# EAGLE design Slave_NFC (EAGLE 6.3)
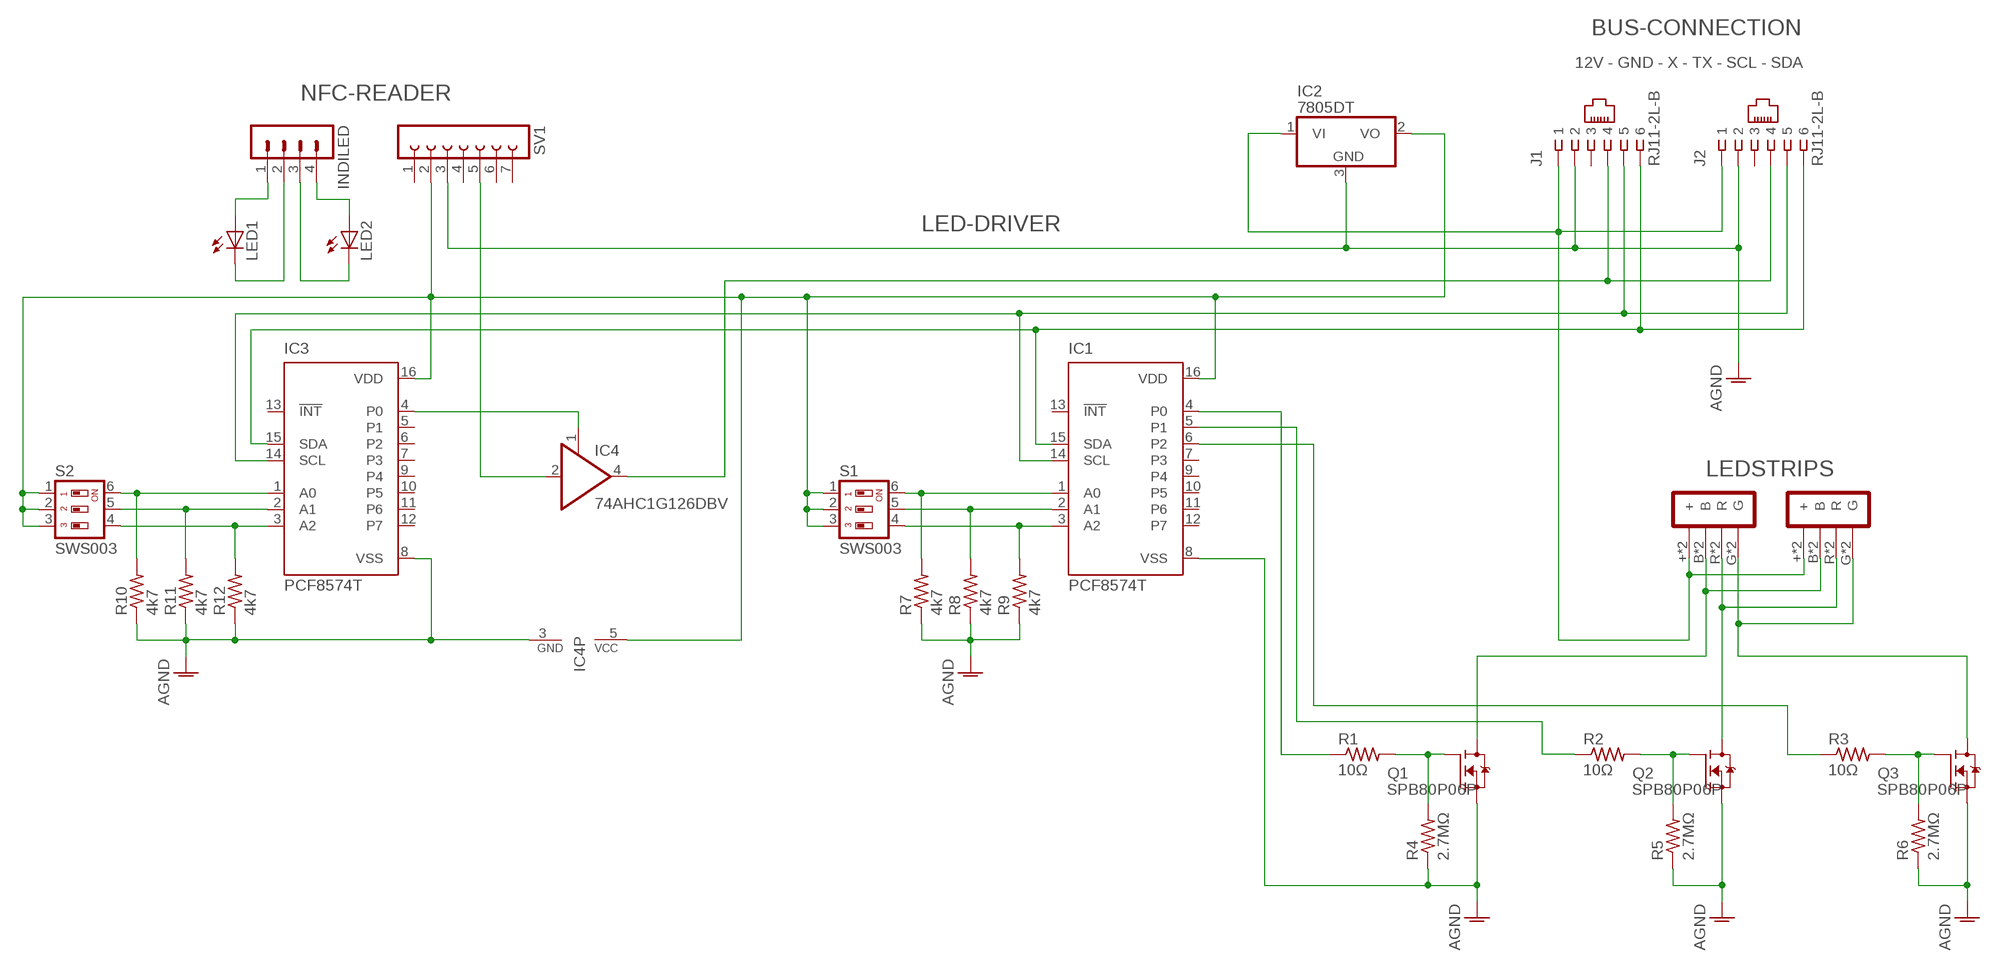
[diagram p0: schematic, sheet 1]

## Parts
IC1  PCF8574T  [SO16W]
IC2  7805DT  [TO252]
IC3  PCF8574T  [SO16W]
IC4  74AHC1G126DBV  [SOT23-5]
INDILED  MA04-1  [MA04-1]
J1  RJ11-2L-B  [RJ11-NO_SHIELD]
J2  RJ11-2L-B  [RJ11-NO_SHIELD]
LED1  LEDB152  [Q62902-B152]
LED2  LEDB152  [Q62902-B152]
Q1  SPB80P06P  [TO263]
Q2  SPB80P06P  [TO263]
Q3  SPB80P06P  [TO263]
R1  10Ω  R-US_R0402  [R0402]
R2  10Ω  R-US_R0402  [R0402]
R3  10Ω  R-US_R0402  [R0402]
R4  2.7MΩ  R-US_R0402  [R0402]
R5  2.7MΩ  R-US_R0402  [R0402]
R6  2.7MΩ  R-US_R0402  [R0402]
R7  4k7  R-US_R0402  [R0402]
R8  4k7  R-US_R0402  [R0402]
R9  4k7  R-US_R0402  [R0402]
R10  4k7  R-US_R0402  [R0402]
R11  4k7  R-US_R0402  [R0402]
R12  4k7  R-US_R0402  [R0402]
S1  SWS003  [SMS-003]
S2  SWS003  [SMS-003]
SV1  FE07-1  [FE07]
U$1  LED_S  [LED_P]
U$2  LED_S  [LED_P]

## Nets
AGND: IC1.8(VSS) IC2.3(GND) IC3.8(VSS) IC4.3(GND) J1.2 J2.2 Q1.2(D) Q2.2(D) Q3.2(D) R4.1 R5.1 R6.1 R7.1 R8.1 R9.1 R10.1 R11.1 R12.1 SV1.3
N$1: IC1.15(SDA) IC3.15(SDA) J1.6 J2.6
N$2: IC4.4(O) J1.4 J2.4
N$3: IC1.14(SCL) J1.5 J2.5
N$4: Q1.1(G) R1.2 R4.2
N$5: Q2.1(G) R2.2 R5.2
N$6: Q3.1(G) R3.2 R6.2
N$7: Q1.3(S) U$1.B U$1.B1(B) U$2.B U$2.B1(B)
N$8: Q2.3(S) U$1.R U$1.R1(R) U$2.R U$2.R1(R)
N$9: Q3.3(S) U$1.G U$1.G1(G) U$2.G U$2.G1(G)
N$10: IC2.1(VI) J1.1 J2.1 U$1.+ U$1.+1(+) U$2.+ U$2.+1(+)
N$11: IC3.1(A0) R10.2 S2.6
N$12: IC1.1(A0) R7.2 S1.6
N$13: IC1.2(A1) R8.2 S1.5
N$14: IC1.3(A2) R9.2 S1.4
N$15: IC3.4(P0) IC4.1(OE)
N$16: IC1.4(P0) R1.1
N$17: IC1.5(P1) R2.1
N$18: IC1.6(P2) R3.1
N$19: IC3.2(A1) R11.2 S2.5
N$20: IC3.3(A2) R12.2 S2.4
N$21: IC1.16(VDD) IC2.2(VO) IC3.16(VDD) IC4.5(VCC) S1.1 S1.2 S1.3 S2.1 S2.2 S2.3 SV1.2
N$22: INDILED.1 LED1.A
N$23: INDILED.4 LED2.A
N$24: INDILED.2 LED1.K(C)
N$25: INDILED.3 LED2.K(C)
N$27: IC4.2(I) SV1.5
Unconnected: IC1.7(P3) IC1.9(P4) IC1.10(P5) IC1.11(P6) IC1.12(P7) IC1.13(!INT) IC3.5(P1) IC3.6(P2) IC3.7(P3) IC3.9(P4) IC3.10(P5) IC3.11(P6) IC3.12(P7) IC3.13(!INT) IC3.14(SCL) J1.3 J2.3 SV1.1 SV1.4 SV1.6 SV1.7

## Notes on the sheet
- BUS-CONNECTION
- 12V - GND - X - TX - SCL - SDA
- NFC-READER
- LED-DRIVER
- LEDSTRIPS

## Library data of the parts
IC1 IC3 = micro-philips:PCF8574: I2C-Bus Remote 8-bit I/O expander http://www.semiconductors.philips.com/acrobat_download/datasheets/PCF8574_4.pdf; MPN: PCF8574T/3,512; OC_FARNELL: 1201255; OC_NEWARK: 70R6870
IC2 = linear:78*: Positive VOLTAGE REGULATOR Source: http://cache.national.com/ds/LM/LM78L05.pdf http://www.fairchildsemi.com/ds/LM/LM7805.pdf
IC4 = 74xx-little-de:74*1G126: Single Bus Buffer Gate With 3-State Outputs
INDILED = con-lstb:MA04-1: PIN HEADER; OC_FARNELL: unknown; OC_NEWARK: unknown
J1 J2 = con-tycoelectronics:RJ11: CORCOM Modular RJ Jacks No Shield Source: www.tycoelectronics.com .. ENG_DS_1654001_1099_RJ_L_0507.pdf; MF: TYCO ELECTRONICS; MPN: RJ11-2L-B; OC_FARNELL: unknown; OC_NEWARK: 83F4463
LED1 LED2 = led:LED: LED
Q1-Q3 = F3205S:SPB80P06P: SIPMOS (R) Power-Transistor P-Channel, Enhancement mode Source: http://www.infineon.com/upload/Document/cmc_upload/documents/011/3685/SPP80P06P.pdf
R1-R12 = rcl:R-US_: RESISTOR, American symbol
S1 S2 = smd-special:SWS003: SMD Dip Switch 3 pol.
SV1 = con-lsta:FE07-1: FEMALE HEADER; OC_FARNELL: unknown; OC_NEWARK: unknown
U$1 U$2 = Onboard_LEDstrip:LED_S

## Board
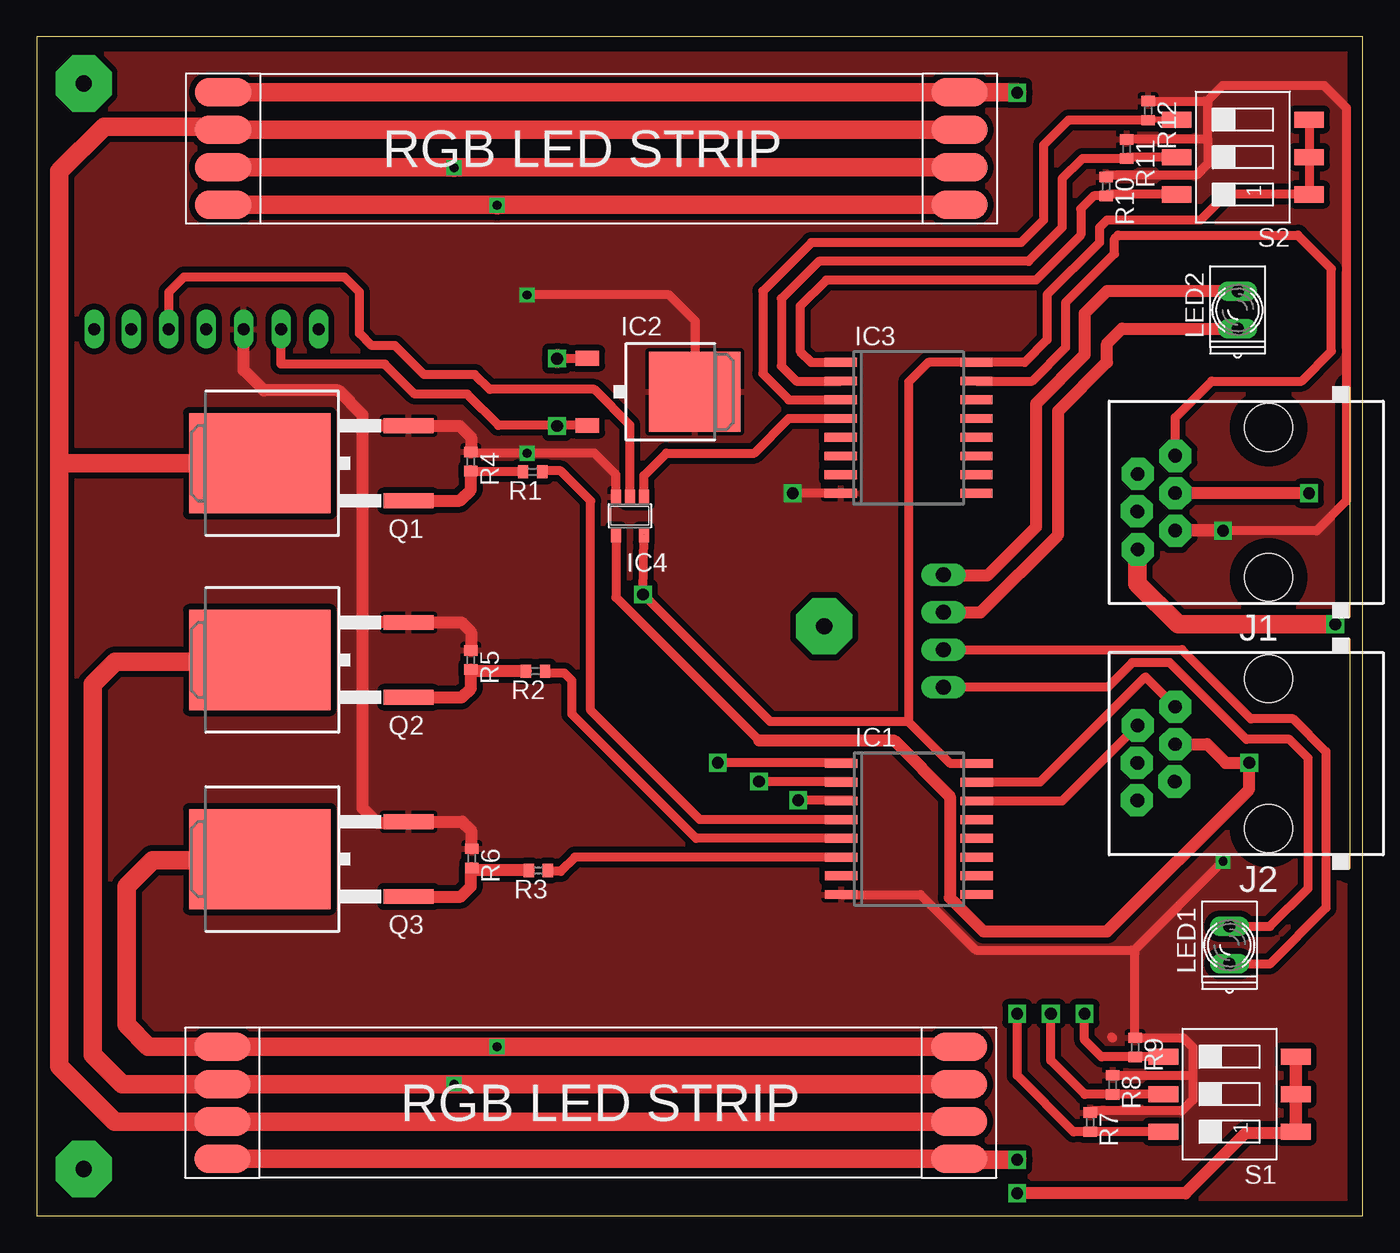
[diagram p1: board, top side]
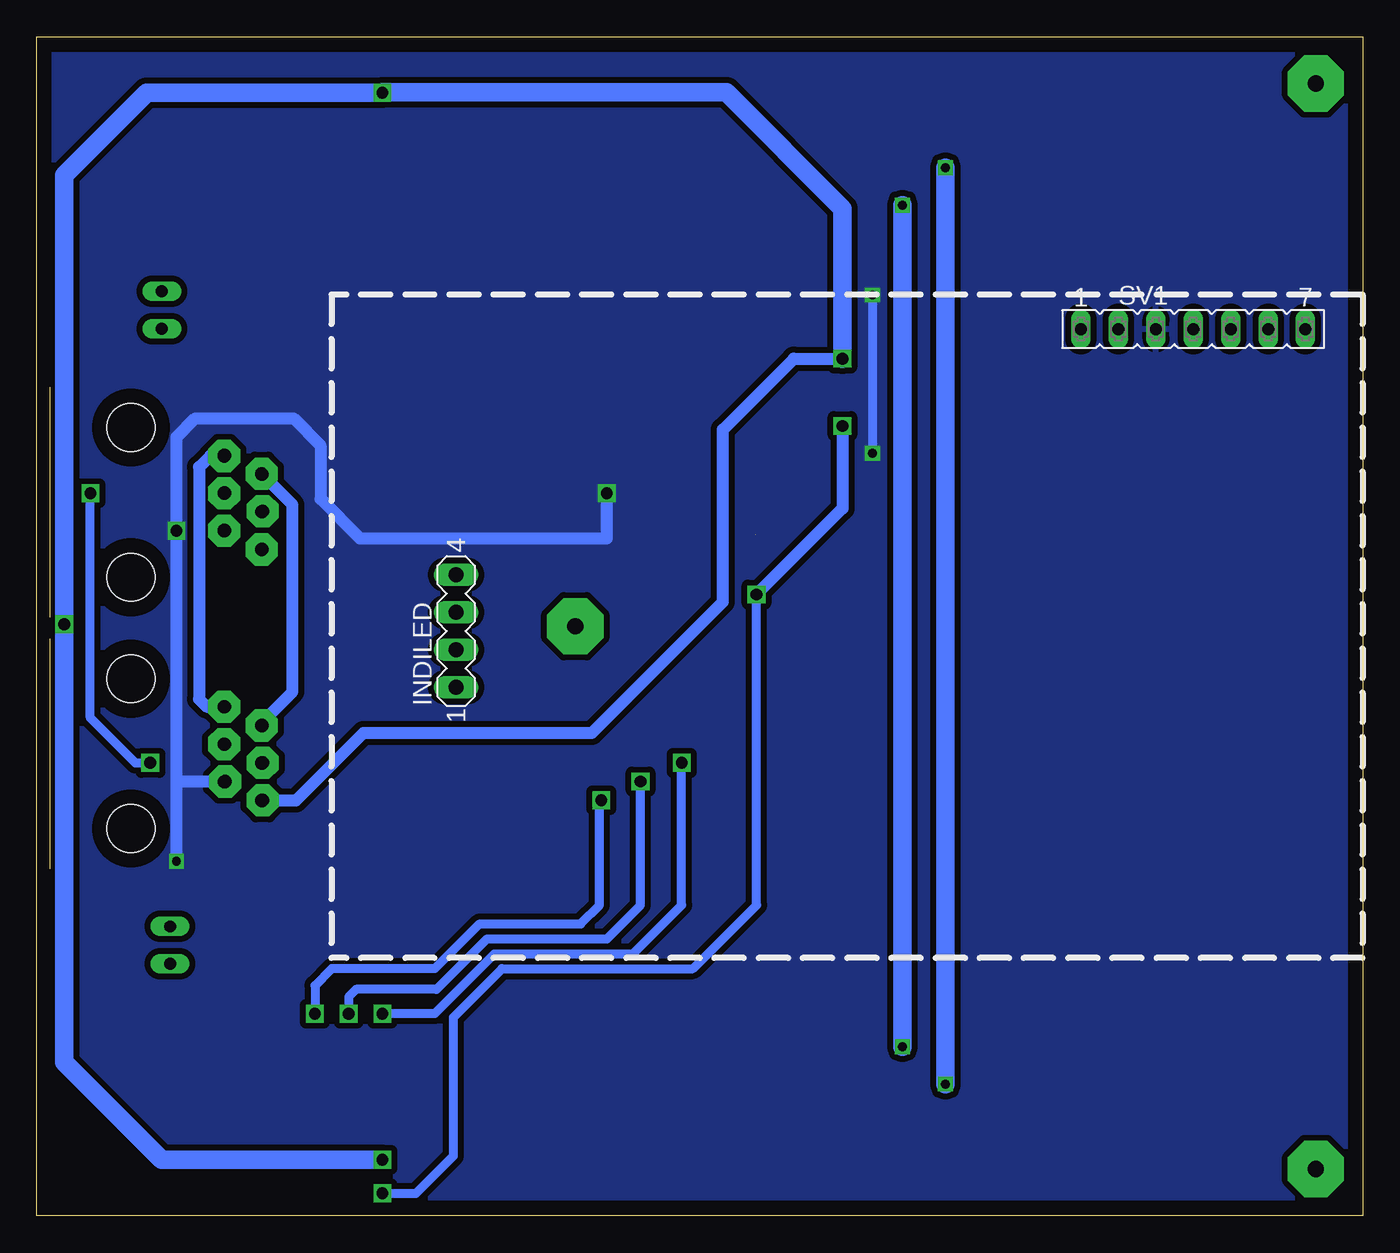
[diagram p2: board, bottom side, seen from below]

Size 90 x 80 mm. Coordinates in mm from the lower left corner, seen from the top.
Outline: 0,0 90,0 90,80 0,80 0,0
Copper layers (1*16): Top 0.035mm / dielectric 1.5mm / Bottom 0.035mm
Design rules "default": minimum track width 10mil, minimum drill 24mil, track to track 8mil, track to pad 8mil, pad to pad 8mil, via to via 8mil, smd to smd 8mil, copper to edge 40mil, drill to drill 8mil, minimum pad ring 10mil, minimum via ring 8mil, stop-mask expansion 4mil, vias tented up to drill 0mil, thermal gap 10mil

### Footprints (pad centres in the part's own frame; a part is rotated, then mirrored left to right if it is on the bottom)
SO16W = smd 0.6 x 2.2: 1 -4.445,-4.6; 2 -3.175,-4.6; 3 -1.905,-4.6; 4 -0.635,-4.6; 5 0.635,-4.6; 6 1.905,-4.6; 7 3.175,-4.6; 8 4.445,-4.6; 9 4.445,4.6; 10 3.175,4.6; 11 1.905,4.6; 12 0.635,4.6; 13 -0.635,4.6; 14 -1.905,4.6; 15 -3.175,4.6; 16 -4.445,4.6
TO252 = smd 1 x 1.6: 1 -2.28,-4.8; 2 2.28,-4.8 | smd 5.4 x 6.2: 3 0,2.5
SOT23-5 = smd 0.69 x 0.99: 1 -0.95,-1.29; 2 0,-1.29; 3 0.95,-1.29; 4 0.95,1.3; 5 -0.95,1.3
MA04-1 = drill 1.016 long: 1 -3.81,0; 2 -1.27,0; 3 1.27,0; 4 3.81,0
RJ11-NO_SHIELD = drill 0.9 pad 1.4: 1 -3.175,8.89; 2 -1.905,6.35; 3 -0.635,8.89; 4 0.635,6.35; 5 1.905,8.89; 6 3.175,6.35 | hole 3.251: -5.08,0; 5.08,0
Q62902-B152 = drill 0.813 long: A 1.27,0; K -1.27,0
TO263 = smd 1 x 3.4: 1 -2.54,-6.6; 2 2.54,-6.6 | smd 6.8 x 9.6: 3 0,3.5
R0402 = smd 0.7 x 0.9: 1 -0.65,0; 2 0.65,0
SMS-003 = smd 1.092 x 2.007: 1 -2.54,-4.496; 2 0,-4.496; 3 2.54,-4.496; 4 2.54,4.496; 5 0,4.496; 6 -2.54,4.496
FE07 = drill 0.813 long: 1 -7.62,0; 2 -5.08,0; 3 -2.54,0; 4 0,0; 5 2.54,0; 6 5.08,0; 7 7.62,0
LED_P = smd 3.81 x 1.93: + -24.13,3.81; +1 25.87,3.81; B -24.13,1.27; B1 25.87,1.27; G -24.13,-3.81; G1 25.87,-3.81; R -24.13,-1.27; R1 25.87,-1.27

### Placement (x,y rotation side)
IC1  59.2,26.25 270 top
IC2  42.17,55.91 270 top
IC3  59.18,53.47 270 top
IC4  40.26,47.5 180 top
INDILED  61.54,39.68 90 bottom
J1  83.61,48.41 90 top
J2  83.61,31.36 90 top
LED1  80.96,18.36 90 top
LED2  81.51,61.47 90 top
Q1  18.63,51.06 90 top
Q2  18.64,37.72 90 top
Q3  18.64,24.2 90 top
R1  33.66,50.48 180 top
R2  33.85,36.96 180 top
R3  34.04,23.43 180 top
R4  29.46,51.18 270 top
R5  29.46,37.72 270 top
R6  29.53,24.26 270 top
R7  71.5,6.35 270 top
R8  73.03,8.89 270 top
R9  74.55,11.43 270 top
R10  72.58,69.85 270 top
R11  73.98,72.39 270 top
R12  75.44,74.99 270 top
S1  80.96,8.26 90 top
S2  81.87,71.84 90 top
SV1  11.5,60.17 0 bottom
U$1  36.78,72.42 0 top
U$2  38.47,7.67 180 top

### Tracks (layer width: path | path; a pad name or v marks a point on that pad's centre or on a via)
AGND  (via drill 0.6, 0.8)
  Top 0.406: 72.58,70.61 R10.1
  Top 0.61: R12.1 79.3,75.64 79.5,75.44 | 79.5,73.04 R11.1 | 79.5,73.04 79.5,71.37 78.74,70.61 72.69,70.61 R10.1 | 79.5,73.04 79.5,75.44 | v80.52,46.48 86.87,46.48 88.9,48.51 88.9,75.18 87.38,76.71 80.52,76.71 79.5,75.69 79.5,75.44 | 78.49,9.4 78.49,11.43 77.84,12.08 R9.1 74.55,17.84 74.36,18.03 | 78.49,9.4 78.49,7.87 77.72,7.11 71.61,7.11 R7.1 | R8.1 78.34,9.54 78.49,9.4 | 73.01,12.08 72.96,12.13 | IC4.3 39.31,50.29 37.85,51.75 v33.27,51.75 29.54,51.75 R4.1 | IC1.8 59.99,21.8 63.75,18.03 74.49,18.03 v80.52,24.07 | IC2.3 44.7,55.91 44.7,60.71 42.93,62.48 v33.27,62.48 | IC3.8 v51.31,49.02
  Top 0.813: R6.1 29.46,24.97 29.46,26.16 28.88,26.74 Q3.2 25.17,26.67 23.11,26.67 22.1,27.69 22.1,40.13 | R5.1 29.46,39.62 28.83,40.26 Q2.2 22.23,40.26 22.1,40.13 | R4.1 29.46,52.83 28.69,53.6 Q1.2 22.11,53.6 22.1,52.83 | 22.1,52.83 22.1,40.13 | 22.1,52.83 22.1,54.36 20.45,56.01 15.43,56.01 14.03,57.4 SV1.3 | IC2.3 44.96,56.21 | v80.52,46.48 77.28,46.48 | v80.5,46.51 J1.2
  Bottom 0.61: v33.27,62.48 v33.27,51.75
  Bottom 0.813: 80.52,29.46 v80.52,46.48 | J2.2 80.51,29.45 80.52,29.46 | v80.5,46.51 v80.52,46.48 | v80.52,46.48 80.52,52.83 79.25,54.1 72.58,54.1 70.74,52.26 70.74,48.64 68.07,45.97 51.31,45.97 v51.31,49.02 | v80.52,24.07 80.52,29.46
  pour Bottom (isolate 0.406): 0.13,80.01 89.98,80.01 89.98,0 0,0 0,80.01
  pour Top (isolate 0.406): 0,80.01 89.92,80.01 89.92,0 0,0
N$1  (via drill 0.9 pad 2.18)
  Top 0.61: IC3.15 67.56,56.64 69.85,58.93 69.85,61.98 73.15,65.28 73.15,66.29 73.41,66.55 85.6,66.55 87.88,64.26 87.88,58.67 85.85,56.64 79.76,56.64 77.28,54.17 77.28,51.56 J1.6 | v77.27,34.54 J2.6 | v77.28,34.54 75.25,36.58 68.09,29.42 IC1.15
  Bottom 0.813: J2.6 v77.27,34.54 v77.28,34.54 78.49,34.54 78.99,35.05 78.99,50.8 78.21,51.59 J1.6
N$2  (via drill 0.8, 0.9 pad 2.18)
  Top 0.61: IC4.4 39.31,41.97 49.02,32.26
  Top 0.813: 49.02,32.26 58.17,32.26 61.98,28.45 61.98,21.59 64.26,19.3 72.64,19.3 82.3,28.96 v82.3,30.73 80.71,30.73 79.44,32 v77.28,32 J2.4 | v86.36,49.02 77.28,49.02 J1.4
  Bottom 0.61: v86.36,49.02 86.36,33.78 83.31,30.73 v82.3,30.73
  Bottom 0.813: 77.28,49.02 J1.4
N$3
  Top 0.61: IC1.14 69.61,28.15 J2.5
  Bottom 0.813: J2.5 74.72,33.48 72.64,35.56 72.64,48.24 J1.5
N$4
  Top 0.61: R1.2 29.51,50.48
  Top 0.813: Q1.1 28.71,48.52 29.46,49.28 R4.2 29.51,50.48
N$5
  Top 0.813: Q2.1 28.83,35.18 29.46,35.81 R5.2 29.58,36.96 R2.2
N$6
  Top 0.813: Q3.1 28.77,21.66 29.46,22.35 29.46,23.54 R6.2 29.7,23.43 R3.2
N$7
  Top 1.27: U$2.B U$2.B1 5.29,6.4 1.52,10.16 1.52,51.05 | 12.06,73.69 U$1.B 13.21,73.69 | U$1.B1 13.21,73.69 | 1.52,51.05 1.52,70.87 4.57,73.91 12.98,73.91 13.21,73.69 | Q1.3 1.53,51.06 1.52,51.05
N$8  (via drill 0.6)
  Top 1.27: U$2.R 62.6,9.21 61.91,9.21 61.91,8.94 28.83,8.94 v28.32,8.94 U$2.R1 5.79,8.94 3.81,10.92 3.81,36.07 5.33,37.59 11.68,37.59 11.94,37.34 11.71,37.34 Q2.3 | U$1.R1 U$1.R 28.3,71.14 v28.32,71.12
  Bottom 1.27: v28.32,71.12 v28.32,8.94
N$9  (via drill 0.6)
  Top 1.27: U$2.G v31.24,11.48 30.99,11.48 U$2.G1 7.57,11.48 6.1,12.95 6.1,22.35 7.87,24.13 15.07,24.13 Q3.3 | U$1.G1 U$1.G 31.22,68.61 v31.24,68.58
  Bottom 1.27: v31.24,68.58 v31.24,11.48
N$10  (via drill 0.8)
  Top 0.61: 35.34,58.2 IC2.1
  Top 1.27: U$2.+1 U$2.+ 62.65,3.81 v66.55,3.81 | U$1.+ U$1.+1 66.52,76.22 v66.55,76.2 | J1.1 74.72,42.88 77.47,40.13 v88.14,40.13 | 35.34,58.2 v35.31,58.17
  Bottom 0.813: J2.1 72.4,28.18 67.82,32.77 52.32,32.77 43.43,41.66 43.43,53.34 38.61,58.17 v35.31,58.17
  Bottom 1.27: v66.55,3.81 81.53,3.81 88.14,10.41 v88.14,40.13 88.14,70.61 82.55,76.2 v66.55,76.2 66.52,76.22 43.18,76.22 35.31,68.35 v35.31,58.17
N$11
  Top 0.406: 72.58,69.3 R10.2
  Top 0.61: S2.6 72.68,69.3 R10.2 71.74,69.2 70.87,68.33 70.87,66.55 67.82,63.5 53.59,63.5 51.82,61.72 51.82,58.67 52.58,57.91 IC3.1
N$12  (via drill 0.8)
  Top 0.61: S1.6 71.52,5.71 R7.2 70.37,5.7 66.55,9.53 v66.55,13.72 | IC1.1 55.38,30.73 v46.23,30.73
  Bottom 0.61: v66.55,13.72 62.99,13.72 58.93,17.78 49.53,17.78 46.23,21.08 v46.23,30.73
N$13  (via drill 0.8)
  Top 0.61: S1.5 73.04,8.26 R8.2 71.14,8.24 68.83,10.54 v68.83,13.72 | IC1.2 55.38,29.46 v49.02,29.46
  Bottom 0.61: v68.83,13.72 68.83,14.86 68.33,15.37 62.87,15.37 59.44,18.8 51.31,18.8 49.02,21.08 v49.02,29.46
N$14  (via drill 0.8)
  Top 0.61: S1.4 74.56,10.79 R9.2 72.28,10.78 71.12,11.94 v71.12,13.72 | IC1.3 55.38,28.19 v51.69,28.19
  Bottom 0.61: v71.12,13.72 71.12,15.62 69.98,16.76 62.99,16.76 59.94,19.81 53.09,19.81 51.82,21.08 51.82,28.07 v51.69,28.19
N$15
  Top 0.61: IC4.1 41.21,50.23 42.74,51.75 48.7,51.75 51.05,54.1 IC3.4
N$16
  Top 0.61: IC1.4 45,26.88 37.59,34.29 37.59,48.51 35.56,50.55 34.37,50.55 R1.1
N$17
  Top 0.61: IC1.5 44.75,25.61 36.32,34.04 36.32,36.32 35.81,36.83 34.62,36.83 R2.1
N$18
  Top 0.61: IC1.6 36.53,24.34 35.56,23.37 34.75,23.37 R3.1
N$19
  Top 0.406: 73.98,71.84 R11.2
  Top 0.61: S2.5 74.08,71.84 R11.2 70.98,71.74 69.6,70.36 69.6,67.06 67.31,64.77 53.09,64.77 50.55,62.23 50.55,57.66 51.56,56.64 IC3.2
N$20
  Top 0.406: S2.4 75.44,74.38 R12.2
  Top 0.61: R12.2 70.03,74.34 68.33,72.64 68.33,67.56 66.8,66.04 52.58,66.04 49.28,62.74 49.28,57.15 51.05,55.37 IC3.3
N$21  (via drill 0.8)  (1 unrouted)
  Top 0.61: S2.3 S2.2 S2.1 80.73,69.3 78.99,67.56 72.64,67.56 72.14,67.06 72.14,66.04 68.58,62.48 68.58,59.44 67.06,57.91 IC3.16 60.52,57.91 59.18,56.58 59.18,33.53 | IC2.2 35.31,53.63 | 35.31,53.63 v35.31,53.59 | 35.31,53.63 31.33,53.63 29.21,55.75 25.65,55.75 23.62,57.78 16.57,57.78 SV1.2 | IC4.5 v41.15,42.16 49.78,33.53 59.18,33.53 | IC1.16 62.02,30.69 59.18,33.53
  Top 0.813: 35.35,53.63 v35.31,53.59 | S1.1 S1.2 S1.3 S1.1 85.6,5.59 82.04,5.59 77.98,1.52 v66.55,1.52
  Bottom 0.61: v66.55,1.52 64.26,1.52 61.72,4.06 61.72,13.46 58.42,16.76 45.47,16.76 41.15,21.08 v41.15,42.16
  Bottom 0.813: v35.31,53.59 35.31,48.01 v41.15,42.16
N$22
  Top 0.61: LED1.A 83.7,19.63 86.3,22.23 86.3,31.05 85.03,32.32 82.11,32.32 76.9,37.53 74.36,37.53 72.71,35.88 INDILED.1
N$23
  Top 0.813: LED2.A 72.64,62.74 71.12,61.21 71.12,58.42 67.82,55.12 67.82,46.74 64.52,43.43 61.6,43.43 INDILED.4
N$24
  Top 0.61: INDILED.2 77.73,38.41 82.42,33.72 85.28,33.72 87.5,31.5 87.5,20.89 83.69,17.08 LED1.K
N$25
  Top 0.813: INDILED.3 64.06,40.95 69.34,46.23 69.34,54.61 72.64,57.91 72.64,59.18 73.66,60.2 LED2.K
N$27
  Top 0.61: IC4.2 40.26,53.66 37.85,56.07 30.73,56.07 29.72,57.09 26.29,57.09 24.32,59.05 22.73,59.05 21.91,59.88 21.91,62.67 20.89,63.69 9.97,63.69 8.95,62.67 SV1.5
N$28  (via drill 0.9 pad 2.18)
  other vias: 74.74,33.27
N$29  (via drill 0.9 pad 2.18)
  other vias: 74.68,30.73
N$30  (via drill 0.9 pad 2.18)
  other vias: 77.22,29.46
N$31  (via drill 0.9 pad 2.18)
  other vias: 74.68,28.19
N$32  (via drill 0.9 pad 2.18)
  other vias: 74.74,50.36
N$33  (via drill 0.9 pad 2.18)
  other vias: 74.68,47.82
N$34  (via drill 0.9 pad 2.18)
  other vias: 74.74,45.21
N$35  (via drill 0.9 pad 2.18)
  other vias: 77.28,46.48
N$36  (via drill 0.9 pad 2.18)
  other vias: 77.28,49.02
N$37  (via drill 0.9 pad 2.18)
  other vias: 77.28,51.56
N$38  (via drill 1.1 pad 3.81)
  other vias: 3.17,76.83
N$39  (via drill 1.1 pad 3.81)
  other vias: 3.17,3.17
N$40  (via drill 1.1 pad 3.81)
  other vias: 53.45,40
